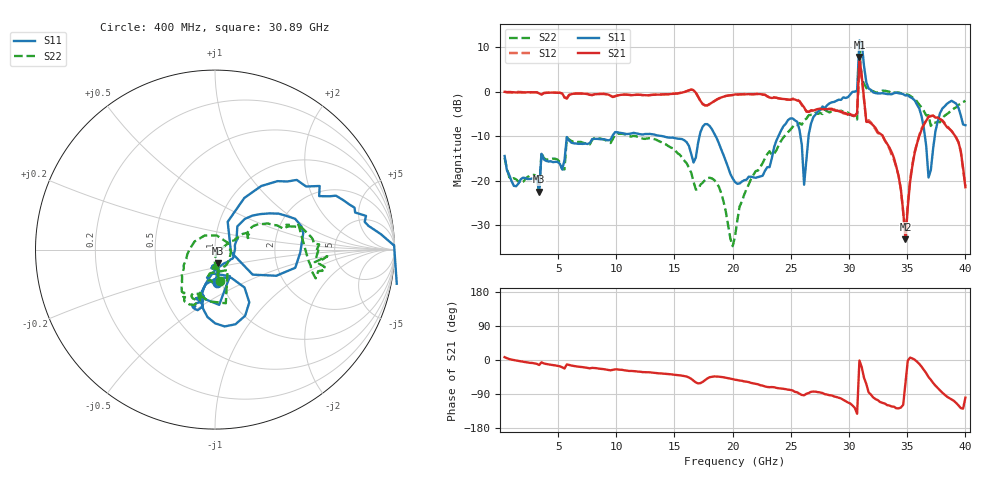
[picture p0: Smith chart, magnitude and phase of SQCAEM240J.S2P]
! Network Analyzer HP8722ES.07.66: Jul 25, 2000 Serial No. US39175408
! 27 Oct 2004  08:49:47
! Frequency  S11  S21  S12  S22
# HZ  S  DB R  50
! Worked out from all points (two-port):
!   201 points, 400 MHz to 40 GHz, reference 50 ohm
!   highest |S21| = 7.77 dB at 30.89 GHz (marker M1); lowest = -33.2 dB at 34.85 GHz (marker M2)
!   |S21| within 3 dB of the highest: 30.84 GHz to 31.03 GHz (189.9 MHz wide, 0.614 % of centre)
!   lowest |S11| = -22.5 dB at 3.37 GHz (marker M3), VSWR 1.16, Z = 50.9 - j7.55 ohm
!   |S11| at or under -10 dB: start of sweep to 9.661 GHz; 13.94 GHz to 17.15 GHz (3.219 GHz wide, 20.7 % of centre); 18.53 GHz to 23.93 GHz (5.401 GHz wide, 25.4 % of centre)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
!   |S22| runs from -34.7 to 9.2 dB; largest |S21 - S12| = 1.1
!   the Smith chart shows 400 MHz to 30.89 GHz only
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4e8  -14.47 -85.8  -0.06 7.5  -0.00 8.8  -14.89 -80.2
3.37e9  -22.48 -78.7  -0.40 -13.2  -0.42 -13.5  -22.61 -81.3
3.568e9  -13.98 -88.7  -0.67 -6.3  -0.64 -6.7  -13.64 -83.4
7.132e9  -11.75 -109.5  -0.44 -18.8  -0.49 -19.5  -11.47 -109.4
1.3666e10  -9.89 -109.7  -0.68 -35.2  -0.64 -35.5  -11.13 -132.0
1.6636e10  -15.94 -87.5  0.32 -54.6  0.34 -55.1  -20.23 126.6
1.7824e10  -7.30 -82.8  -3.09 -48.8  -3.09 -49.4  -19.46 -53.7
2.02e10  -20.31 -72.3  -0.64 -52.1  -0.72 -52.3  -32.60 0.1
2.515e10  -6.02 10.5  -1.71 -80.4  -1.57 -81.7  -7.95 16.8
2.614e10  -20.91 -8.6  -3.53 -93.0  -3.76 -94.2  -6.45 15.5
2.6932e10  -5.74 47.6  -4.26 -83.2  -4.17 -84.7  -5.17 3.7
3.0694e10  0.26 -10.6  -4.81 -141.9  -4.79 -141.0  -6.27 18.4
3.0892e10  11.50 4.5  7.77 -1.3  4.76 -26.4  9.20 -68.8
3.109e10  10.99 2.8  3.60 -18.7  3.24 -20.1  3.04 -31.6
3.1288e10  5.76 -27.1  -1.72 -47.0  -1.93 -48.5  1.72 -20.7
3.1684e10  0.69 -31.4  -6.81 -85.4  -6.42 -86.3  0.21 -20.1
3.3466e10  -0.58 -42.3  -12.55 -120.0  -12.77 -119.8  -0.01 -32.2
3.4852e10  -0.87 -60.5  -33.22 -59.3  -32.49 -49.1  -0.63 -46.9
3.5644e10  -1.97 -78.4  -13.75 0.8  -13.47 1.5  -1.53 -58.1
3.6832e10  -19.30 -99.7  -5.68 -45.0  -5.57 -46.2  -5.29 -63.0
3.802e10  -3.81 9.4  -6.53 -86.3  -6.46 -87.6  -5.91 -38.9
4e10  -7.55 6.2  -21.49 -99.4  -21.19 -96.5  -2.05 -45.8
